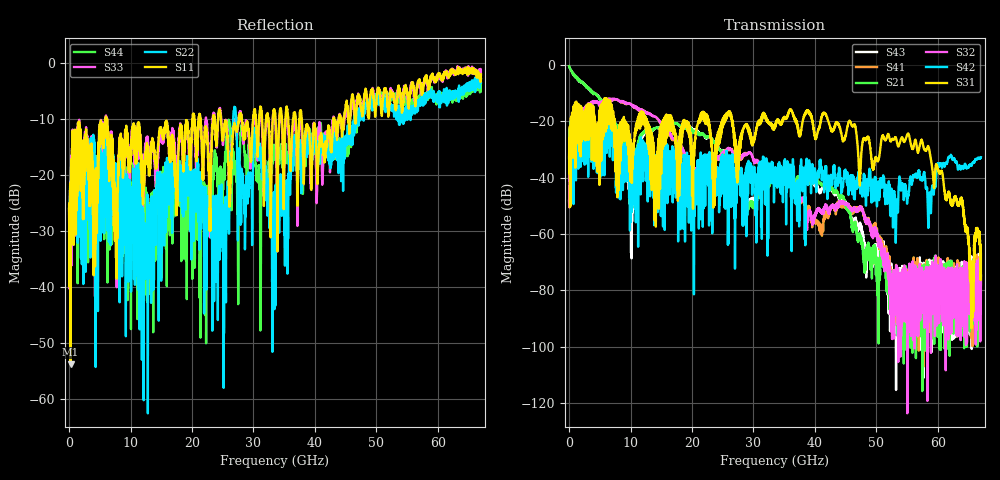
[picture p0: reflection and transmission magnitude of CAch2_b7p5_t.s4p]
!Agilent Technologies,N5247A,US51170199,A.09.90.13
!Agilent N5247A: A.09.90.13
!Date: Tuesday, October 23, 2018 13:54:19
!Correction: S11(Full 4 Port(1,2,3,4))
!S12(Full 4 Port(1,2,3,4))
!S13(Full 4 Port(1,2,3,4))
!S14(Full 4 Port(1,2,3,4))
!S21(Full 4 Port(1,2,3,4))
!S22(Full 4 Port(1,2,3,4))
!S23(Full 4 Port(1,2,3,4))
!S24(Full 4 Port(1,2,3,4))
!S31(Full 4 Port(1,2,3,4))
!S32(Full 4 Port(1,2,3,4))
!S33(Full 4 Port(1,2,3,4))
!S34(Full 4 Port(1,2,3,4))
!S41(Full 4 Port(1,2,3,4))
!S42(Full 4 Port(1,2,3,4))
!S43(Full 4 Port(1,2,3,4))
!S44(Full 4 Port(1,2,3,4))
!S4P File: Measurements: <S11,S12,S13,S14>,
!<S21,S22,S23,S24>,
!<S31,S32,S33,S34>,
!<S41,S42,S43,S44>:
# Hz S  dB  R 50
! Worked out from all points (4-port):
!   6701 points, 10 MHz to 67 GHz, reference 50 ohm
!   strongest paths, dB at 10 MHz, 16.76 GHz, 33.51 GHz, 50.25 GHz, 67 GHz:
!     S31: -32.9, -23.2, -21.1, -34.1, -67.1
!     S42: -33.4, -33.8, -39.6, -43.2, -32.8
!     S32: -48.2, -25.7, -38.0, -60.4, -77.7
!     S21: -0.5, -20.8, -41.4, -81.2, -74.8
!     S41: -48.3, -26.1, -38.8, -61.2, -78.1
!     S43: -0.5, -21.1, -41.1, -67.4, -74.7
!   lowest |S11| = -53.8 dB at 250 MHz (marker M1), VSWR 1.00, Z = 50.2 + j0.0697 ohm
!   |S11| at or under -10 dB: start of sweep to 5.976 GHz; 6.099 GHz to 20.07 GHz (13.97 GHz wide, 107 % of centre); 37.86 GHz to 42.98 GHz (5.122 GHz wide, 12.7 % of centre)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
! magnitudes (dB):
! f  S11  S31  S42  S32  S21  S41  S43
! 10 MHz  -26.1  -32.9  -33.4  -48.2  -0.5  -48.3  -0.5
! 250 MHz  -53.8  -27.8  -28.0  -35.9  -1.7  -35.8  -1.7
! 10.15 GHz  -13.7  -36.0  -43.0  -14.2  -35.1  -14.2  -57.1
! 19.59 GHz  -15.6  -23.5  -34.1  -38.2  -22.5  -43.0  -22.1
! 29.42 GHz  -15.0  -24.5  -36.2  -31.2  -49.0  -31.3  -48.0
! 55.12 GHz  -6.7  -24.5  -46.7  -75.8  -77.7  -80.8  -87.0
! 67 GHz  -2.0  -67.1  -32.8  -77.7  -74.8  -78.1  -74.7
